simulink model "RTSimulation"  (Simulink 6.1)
settings: Solver=FixedStepDiscrete  StartTime=0.0  StopTime=inf  RelTol=1e-3
PreLoadFcn:
  | initialize
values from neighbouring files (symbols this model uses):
  actParams = [	bulkModulus   * pressCanon    [Copy of initialize.m]    (also in initialize.m = [bulkModulus	* pressCanon,)
  aLpf = [1]    [randth.m]
  bLpf = [1]    [randth.m]
  displFreq = inf    [initialize.m]
  flowCanon = 1.666667e+04    (= 16666.67)    [Copy of initialize.m]    (also in initialize.m)
  forceCanon = 1    [Copy of initialize.m]    (also in initialize.m)
  forceFreq = inf    [initialize.m]
  friction = 5			 				* 0.155000	 				* 0.00444822 				* area1    (= 2.71252900422)    [initialize.m]
  fsamp = 1 / samplePeriod    (= 1024)    [Copy of initialize.m]    (also in initialize.m; rampth.m = 1 / deltaT; randth.m = 1 / deltaT; rspect.m = 1.0 / tsamp)
  gasConstant = 1.8    [Copy of initialize.m]    (also in initialize.m)
  lengthCanon = 1    [Copy of initialize.m]    (also in initialize.m)
  massCanon = 1e-06    [Copy of initialize.m]    (also in initialize.m)
  maxDispl = ( (stroke2 + endLength2) * lengthCanon)'    [Copy of initialize.m]    (also in initialize.m = 576.2)
  maxOilVolume = volume * (1 - (precharge/supplyPress)^(1/gasConstant))    (= 211.391477114)    [Copy of initialize.m]    (also in initialize.m)
  maxVeloc = ( (maxFlow' * flowCanon ./ (area1 * areaCanon)) / velocCanon)'    [Copy of initialize.m]    (also in initialize.m = (maxFlow * flowCanon / (area1 * areaCanon)) / velocCanon; rampth.m = 2 * maxDispl / (nVeloc * deltaT))
  minDispl = (-(stroke1 + endLength1) * lengthCanon)'    [Copy of initialize.m]    (also in initialize.m = -576.2)
  minVeloc = (-(maxFlow' * flowCanon ./ (area2 * areaCanon)) / velocCanon)'    [Copy of initialize.m]    (also in initialize.m = -(maxFlow * flowCanon / (area2 * areaCanon)) / velocCanon)
  nAct = 5    [Copy of initialize.m]    (also in initialize.m = 1)
  nAdcU = 6    [Copy of initialize.m]    (also in initialize.m = 5)
  nDout = 4    [Copy of initialize.m]    (also in initialize.m)
  nDucU = 2    [Copy of initialize.m]    (also in initialize.m)
  nEncU = 3    [Copy of initialize.m]    (also in initialize.m)
  node = completenodestruct(node)    [Copy of initialize.m]    (also in initialize.m)
  precharge = 3000		 				* 6.894757e-03    (= 20.684271)    [Copy of initialize.m]    (also in initialize.m)
  pumpFlow = 1e20    (= 1e+20)    [Copy of initialize.m]    (also in initialize.m)
  returnPress = 3			 				* 0.1    (= 0.3)    [Copy of initialize.m]    (also in initialize.m)
  samplePeriod = controlPeriod/upsampleFactor    (= 0.0009765625)    [Copy of initialize.m]    (also in initialize.m; viewer.m = eval(getHeaderValue(header, 'DELTA_T')))
  springCanon = 1    [Copy of initialize.m]    (also in initialize.m)
  supplyPress = 280		 				* 0.1    (= 28)    [Copy of initialize.m]    (also in initialize.m)
  velocCanon = 1    [Copy of initialize.m]    (also in initialize.m)
  volume = 15.15		 				+ (  45		 				    * 2		 				   + 30		 				    * 6 )	 				* 5    (= 1365.15)    [Copy of initialize.m]    (also in initialize.m; quake.m = volume / 231.0)
  volumeCanon = 1e+06    (= 1000000)    [Copy of initialize.m]    (also in initialize.m)
  yieldDispl = 1.0    (= 1)    [initialize.m]
undefined symbols (not defined in the file or in its folder): DiscIntNeverNeededParam, dpforceFreq, mass, spring, staticForce
libraries: xpclib x6, simulink x1
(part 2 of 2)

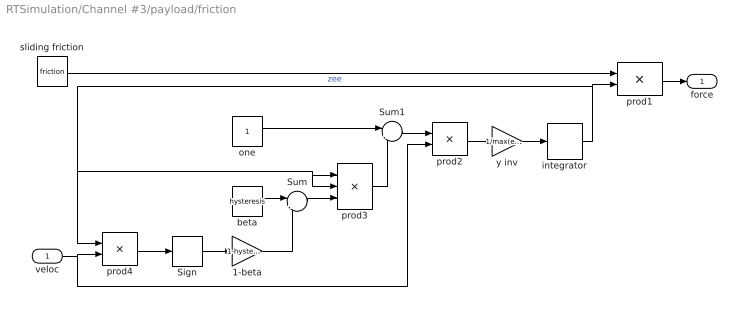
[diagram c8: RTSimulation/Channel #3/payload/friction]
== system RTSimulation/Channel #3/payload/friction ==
  veloc : Inport  Port=1  LatchInput=off
  1-beta : Gain  Gain=1-hysteresis
  Sign : Signum
  Sum : Sum  Inputs=|++
  Sum1 : Sum  Inputs=|+-
  beta : Constant  Value=hysteresis
  integrator : DiscreteIntegrator  SampleTime=-1  LimitOutput=on  UpperSaturationLimit=1  LowerSaturationLimit=-1  ICPrevOutput=DiscIntNeverNeededParam  ICPrevScaledInput=DiscIntNeverNeededParam
  one : Constant
  prod1 : Product
  prod2 : Product
  prod3 : Product  Inputs=3
  prod4 : Product
  sliding friction : Constant  Value=friction
  y inv : Gain  Gain=1/max(eps, yieldDispl)
  force : Outport
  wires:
  integrator/1 -> prod3/2, prod3/1, prod4/1, prod1/2  "zee"
  y inv/1 -> integrator/1
  prod2/1 -> y inv/1
  Sum1/1 -> prod2/1
  prod3/1 -> Sum1/2
  one/1 -> Sum1/1
  Sum/1 -> prod3/3
  beta/1 -> Sum/1
  1-beta/1 -> Sum/2
  Sign/1 -> 1-beta/1
  prod4/1 -> Sign/1
  veloc/1 -> prod2/2, prod4/2
  prod1/1 -> force/1
  sliding friction/1 -> prod1/1

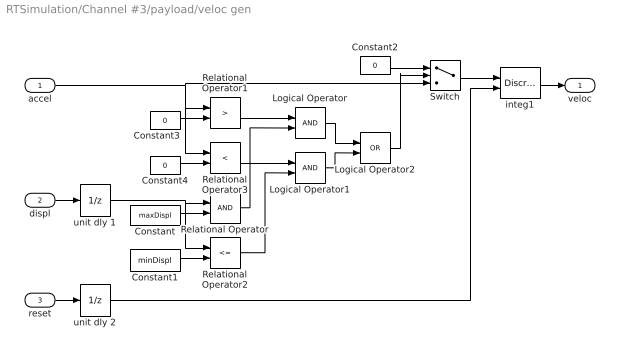
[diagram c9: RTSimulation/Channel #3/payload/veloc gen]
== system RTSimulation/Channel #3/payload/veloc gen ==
  accel : Inport  Port=1  LatchInput=off
  displ : Inport  Port=2  LatchInput=off
  reset : Inport  Port=3  LatchInput=off
  Constant : Constant  Value=maxDispl
  Constant1 : Constant  Value=minDispl
  Constant2 : Constant  Value=0
  Constant3 : Constant  Value=0
  Constant4 : Constant  Value=0
  Logical Operator : Logic
  Logical Operator1 : Logic
  Logical Operator2 : Logic  Operator=OR
  Relational Operator : RelationalOperator
  Relational Operator1 : RelationalOperator  Operator=>
  Relational Operator2 : RelationalOperator  Operator=<=
  Relational Operator3 : RelationalOperator  Operator=<
  Switch : Switch  Threshold=0.5
  integ1 : DiscreteIntegrator  IntegratorMethod=Integration: Backward Euler  ExternalReset=either  SampleTime=-1  LimitOutput=on  UpperSaturationLimit=maxVeloc  LowerSaturationLimit=minVeloc  ICPrevOutput=DiscIntNeverNeededParam  ICPrevScaledInput=DiscIntNeverNeededParam
  unit dly 1 : UnitDelay  SampleTime=-1
  unit dly 2 : UnitDelay  SampleTime=-1
  veloc : Outport
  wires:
  unit dly 1/1 -> Relational Operator2/1, Relational Operator/1
  reset/1 -> unit dly 2/1
  displ/1 -> unit dly 1/1
  Logical Operator1/1 -> Logical Operator2/2
  unit dly 2/1 -> integ1/2
  Switch/1 -> integ1/1
  Logical Operator2/1 -> Switch/2
  Constant2/1 -> Switch/1
  Logical Operator/1 -> Logical Operator2/1
  Relational Operator3/1 -> Logical Operator1/1
  Constant4/1 -> Relational Operator3/2
  Relational Operator1/1 -> Logical Operator/1
  Constant3/1 -> Relational Operator1/2
  accel/1 -> Switch/3, Relational Operator1/1, Relational Operator3/1
  Constant1/1 -> Relational Operator2/2
  Relational Operator2/1 -> Logical Operator1/2
  Relational Operator/1 -> Logical Operator/2
  Constant/1 -> Relational Operator/2
  integ1/1 -> veloc/1

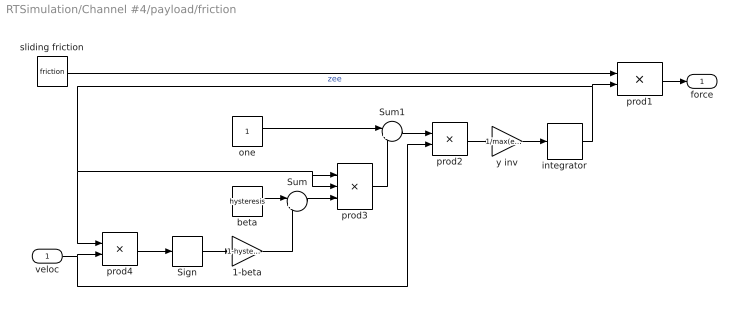
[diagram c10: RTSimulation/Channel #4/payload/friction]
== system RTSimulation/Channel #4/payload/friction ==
  veloc : Inport  Port=1  LatchInput=off
  1-beta : Gain  Gain=1-hysteresis
  Sign : Signum
  Sum : Sum  Inputs=|++
  Sum1 : Sum  Inputs=|+-
  beta : Constant  Value=hysteresis
  integrator : DiscreteIntegrator  SampleTime=-1  LimitOutput=on  UpperSaturationLimit=1  LowerSaturationLimit=-1  ICPrevOutput=DiscIntNeverNeededParam  ICPrevScaledInput=DiscIntNeverNeededParam
  one : Constant
  prod1 : Product
  prod2 : Product
  prod3 : Product  Inputs=3
  prod4 : Product
  sliding friction : Constant  Value=friction
  y inv : Gain  Gain=1/max(eps, yieldDispl)
  force : Outport
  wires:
  sliding friction/1 -> prod1/1
  prod1/1 -> force/1
  veloc/1 -> prod4/2, prod2/2
  prod4/1 -> Sign/1
  Sign/1 -> 1-beta/1
  1-beta/1 -> Sum/2
  beta/1 -> Sum/1
  Sum/1 -> prod3/3
  one/1 -> Sum1/1
  prod3/1 -> Sum1/2
  Sum1/1 -> prod2/1
  prod2/1 -> y inv/1
  y inv/1 -> integrator/1
  integrator/1 -> prod1/2, prod4/1, prod3/1, prod3/2  "zee"

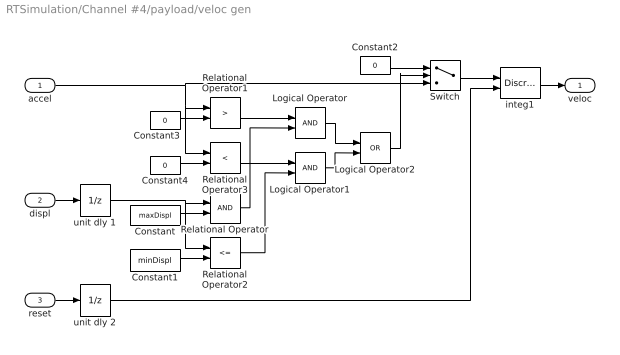
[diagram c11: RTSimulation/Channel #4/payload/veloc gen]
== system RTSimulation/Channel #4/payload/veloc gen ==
  accel : Inport  Port=1  LatchInput=off
  displ : Inport  Port=2  LatchInput=off
  reset : Inport  Port=3  LatchInput=off
  Constant : Constant  Value=maxDispl
  Constant1 : Constant  Value=minDispl
  Constant2 : Constant  Value=0
  Constant3 : Constant  Value=0
  Constant4 : Constant  Value=0
  Logical Operator : Logic
  Logical Operator1 : Logic
  Logical Operator2 : Logic  Operator=OR
  Relational Operator : RelationalOperator
  Relational Operator1 : RelationalOperator  Operator=>
  Relational Operator2 : RelationalOperator  Operator=<=
  Relational Operator3 : RelationalOperator  Operator=<
  Switch : Switch  Threshold=0.5
  integ1 : DiscreteIntegrator  IntegratorMethod=Integration: Backward Euler  ExternalReset=either  SampleTime=-1  LimitOutput=on  UpperSaturationLimit=maxVeloc  LowerSaturationLimit=minVeloc  ICPrevOutput=DiscIntNeverNeededParam  ICPrevScaledInput=DiscIntNeverNeededParam
  unit dly 1 : UnitDelay  SampleTime=-1
  unit dly 2 : UnitDelay  SampleTime=-1
  veloc : Outport
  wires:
  integ1/1 -> veloc/1
  Constant/1 -> Relational Operator/2
  Relational Operator/1 -> Logical Operator/2
  Relational Operator2/1 -> Logical Operator1/2
  Constant1/1 -> Relational Operator2/2
  accel/1 -> Relational Operator3/1, Relational Operator1/1, Switch/3
  Constant3/1 -> Relational Operator1/2
  Relational Operator1/1 -> Logical Operator/1
  Constant4/1 -> Relational Operator3/2
  Relational Operator3/1 -> Logical Operator1/1
  Logical Operator/1 -> Logical Operator2/1
  Constant2/1 -> Switch/1
  Logical Operator2/1 -> Switch/2
  Switch/1 -> integ1/1
  unit dly 2/1 -> integ1/2
  Logical Operator1/1 -> Logical Operator2/2
  displ/1 -> unit dly 1/1
  reset/1 -> unit dly 2/1
  unit dly 1/1 -> Relational Operator/1, Relational Operator2/1
